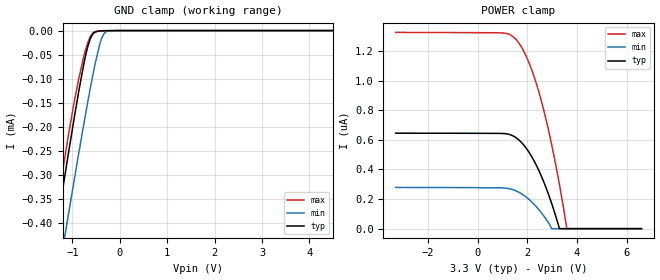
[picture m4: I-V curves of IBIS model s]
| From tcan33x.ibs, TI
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|   s Model
[Model]   s
Model_type   Input
Vinl = 0.66
Vinh = 2.64
|   typ   min   max
|   (nom PVT)   (fast PVT)   (slow PVT)
C_comp   2.903e-13   2.858e-13   3.048e-13
[Model spec]
|subparameter
Vinl   0.66   0.60   0.72
Vinh   2.64   2.40   2.88
| Where nom  PVT is Nominal Process, 3.3V, 27C
|   Fast PVT is Strong Process,  3.6V, -40C
|   Slow PVT is Weak Process,   3V, 150C
[Voltage Range]   3.3   3   3.6
|Junction Temperature
[Temperature Range]   27   150   -40
[Power Clamp Reference]   3.3   3   3.6
[GND Clamp Reference]   0   0   0
[GND Clamp]
|   Voltage   I(typ)   I(min)   I(max)
-3.3V     -1.687mA   -1.742mA   -1.782mA
-1.623V   -597.4uA   -708.9uA   -579.5uA
-1.334V   -413.6uA   -534.2uA   -380.4uA
-1.162V   -305.4uA   -430.6uA   -267.1uA
-1.086V   -258.7uA   -385.7uA   -220.5uA
-874.5mV  -132.9uA   -261.8uA   -105.8uA
-726mV    -55.25uA   -177.6uA   -42.33uA
-620.4mV  -17.21uA   -120.3uA   -12.61uA
-518.1mV  -3.093uA   -68.99uA   -2.122uA
-375mV    -331.7nA   -14.9uA    -440.1nA
-214.5mV  -130.2nA   -435nA     -231nA
6.6V      0A         0A         0A
[POWER Clamp]
|   Voltage   I(typ)   I(min)   I(max)
-3.3V     644.7nA    278.4nA    1.325uA
933.6mV   642.9nA    275.5nA    1.322uA
1.409V    628nA      263.8nA    1.299uA
1.647V    601nA      246.9nA    1.256uA
1.947V    545.4nA    214.5nA    1.168uA
2.241V    467.8nA    170.5nA    1.043uA
2.503V    379.1nA    121nA      901.4nA
2.712V    295.6nA    74.69nA    767.7nA
2.982V    170.5nA    0A         567.9nA
3.297V    0A         0A         296.8nA
3.594V    0A         0A         0A
6.6V      0A         0A         0A
